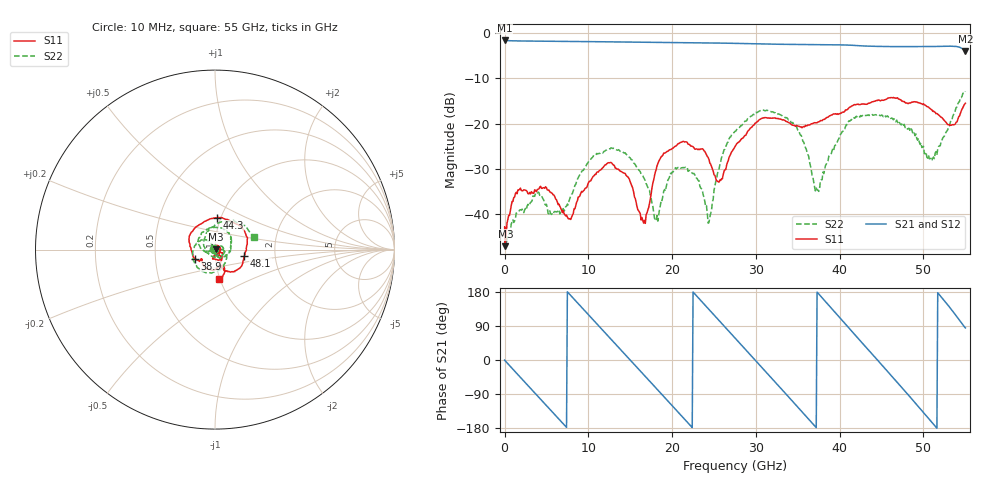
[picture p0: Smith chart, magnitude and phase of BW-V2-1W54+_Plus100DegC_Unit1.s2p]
!Mini-Circuits Laboratory
!S-Parameters
!Type: Fixed Attenuator
!Model: BW-V2-1W54+
!Run / Lot / Date Code: YE0105 / QN2150331 / 2150
!Fixture: N/A, Pressing Arm: N/A
!Network Analyzer: Keysight P9375A;  Serial number: 76634
!Date: 1/25/2022 at 8:22:27 AM
!S/N: Unit# 3 (U1 100°C)
!Tested with: 2 PORT CALIBRATION USING eCAL. DE-EMBEDDED 1.85MM F/F ADAPTER ON PORT 1. TEMP AT 100°C.
!Remark: UNITS TESTED IN 50 OHM SYSTEM, WITHOUT Z-CONVERSION, PORT EXTENSION OFF.
# Hz  S  dB  R  50
!Frequency  S11 dB  S11 Deg  S21 dB  S21 Deg  S12 dB  S12 Deg  S22 dB  S22 Deg
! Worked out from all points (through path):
!   559 points, 10 MHz to 55 GHz, reference 50 ohm
!   highest |S21| = -1.66 dB at 10 MHz (marker M1); lowest = -4.0 dB at 55 GHz (marker M2)
!   group delay of S21, straight-line fit = 67.8 ps
!   lowest |S11| = -47.1 dB at 100 MHz (marker M3), VSWR 1.01, Z = 50.4 + j0.0632 ohm
!   |S11| at or under -10 dB: start of sweep to end of sweep
!   |S22| runs from -46.9 to -12.9 dB; largest |S21 - S12| = 0.0008
!   S11 on the Smith chart (normalised r, x): 10 MHz: 1.01, +0.01; 38.9 GHz: 0.79, -0.08; 44.3 GHz: 0.96, +0.35; 48.1 GHz: 1.38, -0.10; 55 GHz: 0.99, -0.34
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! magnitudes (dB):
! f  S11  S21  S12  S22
! 10 MHz  -43.9  -1.7  -1.7  -46.7
! 100 MHz  -47.1  -1.7  -1.7  -43.5
! 1.8 GHz  -34.5  -1.8  -1.8  -39.1
! 6.8 GHz  -39.1  -1.9  -1.9  -39.5
! 9.2 GHz  -35.0  -1.9  -1.9  -30.6
! 12.7 GHz  -28.6  -2.0  -2.0  -25.4
! 16.6 GHz  -42.0  -2.0  -2.0  -31.9
! 18.4 GHz  -28.4  -2.1  -2.1  -40.1
! 21.6 GHz  -24.0  -2.1  -2.1  -29.6
! 24.5 GHz  -28.7  -2.2  -2.2  -40.7
! 25.7 GHz  -32.5  -2.2  -2.2  -29.1
! 27.6 GHz  -24.8  -2.3  -2.3  -21.7
! 33.5 GHz  -19.4  -2.5  -2.5  -18.7
! 36.7 GHz  -20.0  -2.6  -2.6  -31.4
! 37.4 GHz  -19.7  -2.6  -2.6  -34.7
! 38.9 GHz  -18.2  -2.6  -2.6  -26.9
! 44.3 GHz  -15.0  -3.0  -3.0  -18.0
! 45.9 GHz  -14.3  -3.0  -3.0  -18.4
! 48.1 GHz  -15.6  -3.0  -3.0  -21.3
! 51.1 GHz  -17.3  -3.0  -3.0  -27.7
! 53.5 GHz  -20.2  -2.9  -2.9  -18.4
! 55 GHz  -15.5  -4.0  -4.0  -12.9
